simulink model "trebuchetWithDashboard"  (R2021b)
settings: Solver=VariableStepAuto  StartTime=0.0  StopTime=10.0  MaxStep=1e-4  RelTol=1e-4  AbsTol=1e-5
model workspace (MAT data in the model file):
  alpha0 = 0.920523020141
  finang = 19.6743276335
  lsling = 20
  ppos = 3
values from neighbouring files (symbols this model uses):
  in = repmat(Simulink.SimulationInput(mdl),N,1)    [simulateMultipleTrebuchet.m]    (also in simulateTrebuchet.m = in.setVariable('finang',launchAngle,'workspace',mdl))
  N = 20    [simulateMultipleTrebuchet.m]
undefined symbols (not defined in the file or in its folder): deg, ft, kg, lbm, m, s, X, Y, Z
libraries: sm_lib x33, nesl_utility x6, simulink x1

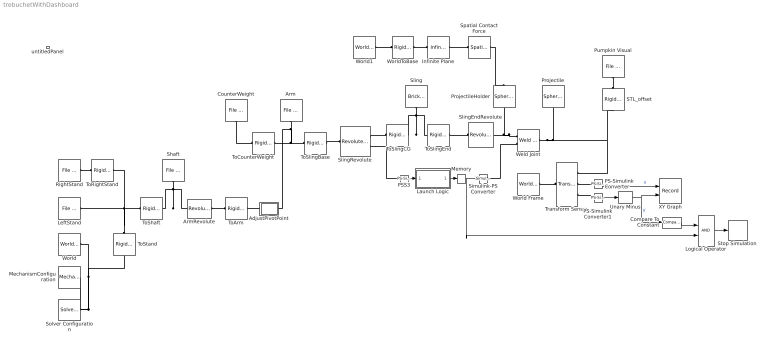
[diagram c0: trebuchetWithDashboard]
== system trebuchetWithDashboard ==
  AdjustPivotPoint : Subsystem
  Arm : sm_lib/Body Elements/File Solid  ExtGeomFileName=arm_prt.stl  UnitType=Custom  ExtGeomFileUnits=in  StepReaderType=HEX  ExportConvexHullGeometry=off  InertiaType=Custom  Mass=1.6  MassUnits=lbm  CenterOfMass=[2.01944889092782 0.231390262424323 -1.93537039141591e-10]  CenterOfMassUnits=in  MomentsOfInertia=[1.99947648053387 238.440492059946 240.01438453116]  MomentsOfInertiaUnits=lbm*in^2  ProductsOfInertia=[0 0 0]  ProductsOfInertiaUnits=lbm*in^2  BasedOnType=Density  Density=800  DensityUnits=kg/(m^3)  DoExposeReferenceFrame=on  SerializedFrames=<Frames/>  GraphicType=FromGeometry  MarkerShape=Sphere  MarkerSize=10  MarkerSizeUnits=m  GraphicVisPropType=SimpleVisualProperties  GraphicDiffuseColor="[0.7137    0.6078    0.2980]"  GraphicSpecularColor=[0.5 0.5 0.5 1.0]  GraphicAmbientColor=[0.15 0.15 0.15 1.0]  GraphicEmissiveColor=[0.0 0.0 0.0 1.0]  GraphicShininess=75  GraphicOpacity=1.0
  ArmRevolute : sm_lib/Joints/Revolute Joint  JointMode=Normal  SenseConstraintForce=off  SenseConstraintForceX=off  SenseConstraintForceY=off  SenseConstraintForceZ=off  SenseConstraintTorque=off  SenseConstraintTorqueX=off  SenseConstraintTorqueY=off  SenseConstraintTorqueZ=off  SenseTotalForce=off  SenseTotalForceX=off  SenseTotalForceY=off  SenseTotalForceZ=off  SenseTotalTorque=off  SenseTotalTorqueX=off  SenseTotalTorqueY=off  SenseTotalTorqueZ=off  CompositeWrenchDir=FollowerOnBase  CompositeWrenchFrame=BaseFrame  EquilibriumPosition=0  EquilibriumPositionUnits=deg  SpringStiffness=0  SpringStiffnessUnits=N*m/deg  DampingCoefficient=0  DampingCoefficientUnits=N*m/(deg/s)  TorqueActuationMode=NoTorque  MotionActuationMode=ComputedMotion  SensePosition=off  SenseVelocity=off  SenseAcceleration=off  SenseTorqueForce=off  SenseLowerLimitTorqueForce=off  SenseUpperLimitTorqueForce=off  LowerLimitSpecify=off  LowerLimitBound=-90  LowerLimitBoundUnits=deg  LowerLimitStiffness=1e4  LowerLimitStiffnessUnits=N*m/deg  LowerLimitDamping=10  LowerLimitDampingUnits=N*m/(deg/s)  LowerLimitTransitionRegionWidth=0.1  LowerLimitTransitionRegionWidthUnits=deg  UpperLimitSpecify=off  UpperLimitBound=90  UpperLimitBoundUnits=deg  UpperLimitStiffness=1e4  UpperLimitStiffnessUnits=N*m/deg  UpperLimitDamping=10  UpperLimitDampingUnits=N*m/(deg/s)  UpperLimitTransitionRegionWidth=0.1  UpperLimitTransitionRegionWidthUnits=deg  PositionTargetSpecify=on  PositionTargetPriority=High  PositionTargetValue=alpha0  PositionTargetValueUnits=rad  VelocityTargetSpecify=off  VelocityTargetPriority=High  VelocityTargetValue=0  VelocityTargetValueUnits=deg/s
  Compare To Constant : simulink/Logic and Bit Operations/Compare To Constant  relop=<=  const=-0.1  OutDataTypeStr=boolean
  CounterWeight : sm_lib/Body Elements/File Solid  ExtGeomFileName=cweight_prt.stl  UnitType=Custom  ExtGeomFileUnits=in  StepReaderType=HEX  ExportConvexHullGeometry=off  InertiaType=Custom  Mass=20  MassUnits=lbm  CenterOfMass=[0 0 0]  CenterOfMassUnits=in  MomentsOfInertia=[180.271839940582 180.271699524682 219.335621261554]  MomentsOfInertiaUnits=lbm*in^2  ProductsOfInertia=[0 0 0]  ProductsOfInertiaUnits=lbm*in^2  BasedOnType=Density  Density=8200  DensityUnits=kg/(m^3)  DoExposeReferenceFrame=on  SerializedFrames=<Frames/>  GraphicType=FromGeometry  MarkerShape=Sphere  MarkerSize=10  MarkerSizeUnits=m  GraphicVisPropType=SimpleVisualProperties  GraphicDiffuseColor=[0.5 0.5 0.5]  GraphicSpecularColor=[0.5 0.5 0.5 1.0]  GraphicAmbientColor=[0.15 0.15 0.15 1.0]  GraphicEmissiveColor=[0.0 0.0 0.0 1.0]  GraphicShininess=75  GraphicOpacity=1.0
  Infinite Plane : sm_lib/Curves and Surfaces/Infinite Plane  GraphicType=Rectangle  GraphicPlaneWidth=5  GraphicPlaneWidthUnits=m  GraphicPlaneHeight=5  GraphicPlaneHeightUnits=m  GraphicVisPropType=SimpleVisualProperties  GraphicDiffuseColor=[1 1 1]  GraphicOpacity=0.25  GraphicSpecularColor=[0.5 0.5 0.5 1.0]  GraphicAmbientColor=[0.15 0.15 0.15 1.0]  GraphicEmissiveColor=[0.0 0.0 0.0 1.0]  GraphicShininess=75
  Launch Logic : Stateflow chart  TreatAsAtomicUnit=on
  LeftStand : sm_lib/Body Elements/File Solid  ExtGeomFileName=upright_prt.stl  UnitType=Custom  ExtGeomFileUnits=in  StepReaderType=HEX  ExportConvexHullGeometry=off  InertiaType=Custom  Mass=5  MassUnits=lbm  CenterOfMass=[0 -6.3095100000000004 0.38968399999999997]  CenterOfMassUnits=in  MomentsOfInertia=[11765.6 43021.699999999997 54038.900000000001]  MomentsOfInertiaUnits=lbm*in^2  ProductsOfInertia=[1161.4200000000001 0 0]  ProductsOfInertiaUnits=lbm*in^2  BasedOnType=Density  Density=1000  DensityUnits=kg/(m^3)  DoExposeReferenceFrame=on  SerializedFrames=<Frames/>  GraphicType=FromGeometry  MarkerShape=Sphere  MarkerSize=10  MarkerSizeUnits=m  GraphicVisPropType=SimpleVisualProperties  GraphicDiffuseColor="[0.5098    0.3216    0.0039]"  GraphicSpecularColor=[0.5 0.5 0.5 1.0]  GraphicAmbientColor=[0.15 0.15 0.15 1.0]  GraphicEmissiveColor=[0.0 0.0 0.0 1.0]  GraphicShininess=75  GraphicOpacity=0.2
  Logical Operator : Logic  AllPortsSameDT=off  OutDataTypeStr=boolean
  MechanismConfiguration : sm_lib/Utilities/Mechanism Configuration  UniformGravity=Constant  GravityVector=[0 32.174 0]  GravityUnits=ft/s^2  LinearizationDelta=0.001  JointModeTransitionNonlinearIterations=2
  Memory : Memory
  PS-Simulink Converter : nesl_utility/PS-Simulink Converter  PhysicalDomain=network_engine_domain  SubClassName=ps_output  LeftPortType=input  RightPortType=output  PseudoPeriodic=off  Frequencies=[]  Unit=inherit  AffineConversion=off
  PS-Simulink Converter1 : nesl_utility/PS-Simulink Converter  PhysicalDomain=network_engine_domain  SubClassName=ps_output  LeftPortType=input  RightPortType=output  PseudoPeriodic=off  Frequencies=[]  Unit=inherit  AffineConversion=off
  PSS3 : nesl_utility/PS-Simulink Converter  PhysicalDomain=network_engine_domain  SubClassName=ps_output  LeftPortType=input  RightPortType=output  PseudoPeriodic=off  Frequencies=[]  Unit=deg  AffineConversion=off
  Projectile : sm_lib/Body Elements/Spherical Solid  GraphicAmbientColor=[0.15 0.15 0.15 1.0]  BasedOnType=Density  CenterOfMass=[0 0 0]  CenterOfMassUnits=m  GraphicDiffuseColor=[0.4 1.0 0.4]  Density=3000*10  DensityUnits=kg/m^3  DoExposeReferenceFrame=on  GraphicEmissiveColor=[0.0 0.0 0.0 1.0]  ExportEntireGeometry=off  SerializedExposedGeometries=<ExposedGeometries/>  SerializedFrames=<Frames/>  MarkerShape=Sphere  MarkerSize=10  GraphicType=FromGeometry  InertiaType=CalculateFromGeometry  Mass=0.074  MassUnits=lbm  MomentsOfInertia=[1 1 1]  MomentsOfInertiaUnits=lbm*in^2  GraphicOpacity=0.2  ProductsOfInertia=[0 0 0]  ProductsOfInertiaUnits=lbm*in^2  GraphicShininess=75  GraphicSpecularColor=[0.5 0.5 0.5 1.0]  SphereRadius=0.624  SphereRadiusUnits=in  GraphicVisPropType=SimpleVisualProperties
  ProjectileHolder : sm_lib/Body Elements/Spherical Solid  GraphicAmbientColor=[0.15 0.15 0.15 1.0]  BasedOnType=Density  CenterOfMass=[0 0 0]  CenterOfMassUnits=m  GraphicDiffuseColor=[1 0.25 0]  Density=3000  DensityUnits=kg/m^3  DoExposeReferenceFrame=on  GraphicEmissiveColor=[0.0 0.0 0.0 1.0]  ExportEntireGeometry=on  SerializedExposedGeometries=<ExposedGeometries><ExposedGeometry><RawGeometryId>entire</RawGeometryId><ExposedGeometryId>G</ExposedGeometryId></ExposedGeometry></ExposedGeometries>  SerializedFrames=<Frames/>  MarkerShape=Sphere  MarkerSize=10  GraphicType=FromGeometry  InertiaType=Custom  Mass=0.001  MassUnits=kg  MomentsOfInertia=[1 1 1]  MomentsOfInertiaUnits=lbm*in^2  GraphicOpacity=1.0  ProductsOfInertia=[0 0 0]  ProductsOfInertiaUnits=lbm*in^2  GraphicShininess=75  GraphicSpecularColor=[0.5 0.5 0.5 1.0]  SphereRadius=0.624  SphereRadiusUnits=in  GraphicVisPropType=SimpleVisualProperties
  Pumpkin Visual : sm_lib/Body Elements/File Solid  ExtGeomFileName=pumpkinskull_earring_remix.stl  UnitType=Custom  ExtGeomFileUnits=cm  StepReaderType=HEX  ExportConvexHullGeometry=off  InertiaType=PointMass  Mass=0  MassUnits=kg  CenterOfMass=[0 0 0]  CenterOfMassUnits=m  MomentsOfInertia=[1 1 1]  MomentsOfInertiaUnits=kg*m^2  ProductsOfInertia=[0 0 0]  ProductsOfInertiaUnits=kg*m^2  BasedOnType=DensityFromFile  Density=1000  DensityUnits=kg/m^3  DoExposeReferenceFrame=on  SerializedFrames=<Frames/>  GraphicType=FromGeometry  MarkerShape=Sphere  MarkerSize=10  GraphicVisPropType=SimpleVisualProperties  GraphicDiffuseColor=[1.0 0.4 0.0]  GraphicSpecularColor=[0.5 0.5 0.5 1.0]  GraphicAmbientColor=[0.15 0.15 0.15 1.0]  GraphicEmissiveColor=[0.0 0.0 0.0 1.0]  GraphicShininess=75  GraphicOpacity=1.0
  RightStand : sm_lib/Body Elements/File Solid  ExtGeomFileName=prt0002_prt.stl  UnitType=Custom  ExtGeomFileUnits=in  StepReaderType=HEX  ExportConvexHullGeometry=off  InertiaType=Custom  Mass=5  MassUnits=lbm  CenterOfMass=[0 -6.3095100000000004 -0.38968399999999997]  CenterOfMassUnits=in  MomentsOfInertia=[11765.6 43021.699999999997 54038.900000000001]  MomentsOfInertiaUnits=lbm*in^2  ProductsOfInertia=[-1161.4200000000001 0 0]  ProductsOfInertiaUnits=lbm*in^2  BasedOnType=Density  Density=1000  DensityUnits=kg/(m^3)  DoExposeReferenceFrame=on  SerializedFrames=<Frames/>  GraphicType=FromGeometry  MarkerShape=Sphere  MarkerSize=10  MarkerSizeUnits=m  GraphicVisPropType=SimpleVisualProperties  GraphicDiffuseColor="[0.5098    0.3216    0.0039]"  GraphicSpecularColor=[0.5 0.5 0.5 1.0]  GraphicAmbientColor=[0.15 0.15 0.15 1.0]  GraphicEmissiveColor=[0.0 0.0 0.0 1.0]  GraphicShininess=75  GraphicOpacity=0.2
  STL_offset : sm_lib/Frames and Transforms/Rigid Transform  TranslationMethod=Cartesian  TranslationStandardOffset=0  TranslationLengthUnit=m  TranslationStandardAxis=+Z  TranslationCartesianOffset=[-1 0 1]  TranslationROffset=0  TranslationROffsetUnits=m  TranslationZOffset=0  TranslationZOffsetUnits=m  TranslationThetaOffset=0  TranslationThetaOffsetUnits=deg  RotationMethod=StandardAxis  RotationAngleUnits=deg  RotationStandardAxis=+X  RotationAngle=-90  RotationArbitraryAxis=[0 0 1]  FollAlignAxisA=+X  BaseAlignAxisA=+Y  FollAlignAxisB=+Y  BaseAlignAxisB=+Z  RotationSequenceAxes=FollowerAxes  RotationSequence=XYX  RotationSequenceAngles=[0 0 0]  RotationSequenceAnglesUnits=deg  RotationMatrix=[1 0 0; 0 1 0; 0 0 1]
  Shaft : sm_lib/Body Elements/File Solid  ExtGeomFileName=shaft1_prt.stl  UnitType=Custom  ExtGeomFileUnits=in  StepReaderType=HEX  ExportConvexHullGeometry=off  InertiaType=Custom  Mass=0.75161  MassUnits=lbm  CenterOfMass=[0 -1.44250608133824e-19 -3.11581313569059e-16]  CenterOfMassUnits=in  MomentsOfInertia=[6.64610546204847 6.64664045415189 0.039282600271159]  MomentsOfInertiaUnits=lbm*in^2  ProductsOfInertia=[0 0 0]  ProductsOfInertiaUnits=lbm*in^2  BasedOnType=Density  Density=7850  DensityUnits=kg/(m^3)  DoExposeReferenceFrame=on  SerializedFrames=<Frames/>  GraphicType=FromGeometry  MarkerShape=Sphere  MarkerSize=10  MarkerSizeUnits=m  GraphicVisPropType=SimpleVisualProperties  GraphicDiffuseColor=[0.5 0.5 0.5]  GraphicSpecularColor=[0.5 0.5 0.5 1.0]  GraphicAmbientColor=[0.15 0.15 0.15 1.0]  GraphicEmissiveColor=[0.0 0.0 0.0 1.0]  GraphicShininess=75  GraphicOpacity=1.0
  Simulink-PS Converter : nesl_utility/Simulink-PS Converter  PhysicalDomain=network_engine_domain  SubClassName=ps_input  LeftPortType=input  RightPortType=output  PseudoPeriodic=off  Frequencies=[]  NoiseDistribution=none  NoiseParameters=[]  Unit=1  AffineConversion=off  FilteringAndDerivatives=provide  SimscapeFilterOrder=1  InputFilterTimeConstant=0.001  UdotUserProvided=0
  Sling : sm_lib/Body Elements/Brick Solid  GraphicAmbientColor=[0.15 0.15 0.15 1.0]  BasedOnType=Density  BrickDimensions=[lsling .05 .05]  BrickDimensionUnits=in  CenterOfMass=[0 0 0]  CenterOfMassUnits=m  GraphicDiffuseColor=[0.0 0 0.0]  Density=1  DensityUnits=kg/(m^3)  DoExposeReferenceFrame=on  GraphicEmissiveColor=[0.0 0.0 0.0 1.0]  ExportEntireGeometry=off  SerializedFrames=<Frames/>  MarkerShape=Sphere  MarkerSize=10  GraphicType=FromGeometry  InertiaType=CalculateFromGeometry  Mass=1  MassUnits=kg  MomentsOfInertia=[1 1 1]  MomentsOfInertiaUnits=kg*m^2  GraphicOpacity=1.0  ProductsOfInertia=[0 0 0]  ProductsOfInertiaUnits=kg*m^2  GraphicShininess=75  GraphicSpecularColor=[0.5 0.5 0.5 1.0]  GraphicVisPropType=SimpleVisualProperties
  SlingEndRevolute : sm_lib/Joints/Revolute Joint  JointMode=Normal  SenseConstraintForce=off  SenseConstraintForceX=off  SenseConstraintForceY=off  SenseConstraintForceZ=off  SenseConstraintTorque=off  SenseConstraintTorqueX=off  SenseConstraintTorqueY=off  SenseConstraintTorqueZ=off  SenseTotalForce=off  SenseTotalForceX=off  SenseTotalForceY=off  SenseTotalForceZ=off  SenseTotalTorque=off  SenseTotalTorqueX=off  SenseTotalTorqueY=off  SenseTotalTorqueZ=off  CompositeWrenchDir=FollowerOnBase  CompositeWrenchFrame=BaseFrame  EquilibriumPosition=0  EquilibriumPositionUnits=deg  SpringStiffness=0  SpringStiffnessUnits=N*m/deg  DampingCoefficient=0  DampingCoefficientUnits=N*m/(deg/s)  TorqueActuationMode=NoTorque  MotionActuationMode=ComputedMotion  SensePosition=off  SenseVelocity=off  SenseAcceleration=off  SenseTorqueForce=off  SenseLowerLimitTorqueForce=off  SenseUpperLimitTorqueForce=off  LowerLimitSpecify=off  LowerLimitBound=-90  LowerLimitBoundUnits=deg  LowerLimitStiffness=1e4  LowerLimitStiffnessUnits=N*m/deg  LowerLimitDamping=10  LowerLimitDampingUnits=N*m/(deg/s)  LowerLimitTransitionRegionWidth=0.1  LowerLimitTransitionRegionWidthUnits=deg  UpperLimitSpecify=off  UpperLimitBound=90  UpperLimitBoundUnits=deg  UpperLimitStiffness=1e4  UpperLimitStiffnessUnits=N*m/deg  UpperLimitDamping=10  UpperLimitDampingUnits=N*m/(deg/s)  UpperLimitTransitionRegionWidth=0.1  UpperLimitTransitionRegionWidthUnits=deg  PositionTargetSpecify=off  PositionTargetPriority=High  PositionTargetValue=-48.6  PositionTargetValueUnits=deg  VelocityTargetSpecify=off  VelocityTargetPriority=High  VelocityTargetValue=0  VelocityTargetValueUnits=deg/s
  SlingRevolute : sm_lib/Joints/Revolute Joint  JointMode=Normal  SenseConstraintForce=off  SenseConstraintForceX=off  SenseConstraintForceY=off  SenseConstraintForceZ=off  SenseConstraintTorque=off  SenseConstraintTorqueX=off  SenseConstraintTorqueY=off  SenseConstraintTorqueZ=off  SenseTotalForce=off  SenseTotalForceX=off  SenseTotalForceY=off  SenseTotalForceZ=off  SenseTotalTorque=off  SenseTotalTorqueX=off  SenseTotalTorqueY=off  SenseTotalTorqueZ=off  CompositeWrenchDir=FollowerOnBase  CompositeWrenchFrame=BaseFrame  EquilibriumPosition=0  EquilibriumPositionUnits=deg  SpringStiffness=0  SpringStiffnessUnits=N*m/deg  DampingCoefficient=0  DampingCoefficientUnits=N*m/(deg/s)  TorqueActuationMode=NoTorque  MotionActuationMode=ComputedMotion  SensePosition=on  SenseVelocity=off  SenseAcceleration=off  SenseTorqueForce=off  SenseLowerLimitTorqueForce=off  SenseUpperLimitTorqueForce=off  LowerLimitSpecify=off  LowerLimitBound=-90  LowerLimitBoundUnits=deg  LowerLimitStiffness=1e4  LowerLimitStiffnessUnits=N*m/deg  LowerLimitDamping=10  LowerLimitDampingUnits=N*m/(deg/s)  LowerLimitTransitionRegionWidth=0.1  LowerLimitTransitionRegionWidthUnits=deg  UpperLimitSpecify=off  UpperLimitBound=90  UpperLimitBoundUnits=deg  UpperLimitStiffness=1e4  UpperLimitStiffnessUnits=N*m/deg  UpperLimitDamping=10  UpperLimitDampingUnits=N*m/(deg/s)  UpperLimitTransitionRegionWidth=0.1  UpperLimitTransitionRegionWidthUnits=deg  PositionTargetSpecify=on  PositionTargetPriority=High  PositionTargetValue=-35  PositionTargetValueUnits=deg  VelocityTargetSpecify=off  VelocityTargetPriority=High  VelocityTargetValue=0  VelocityTargetValueUnits=deg/s
  Solver Configuration : nesl_utility/Solver Configuration  PhysicalDomain=network_engine_domain  SubClassName=solver  LeftPortType=input  RightPortType=generic  Tones=[]  Harmonics=[]  SimulateNoise=off  Profile=off  UseLocalSampling=off  EnableSwitchedLinearOptims=on  FrequencyDomain=off  UseCCode=off  RelTol=0.001  AbsTol=1e-06  MinStep=1e-09  ToWorkspace=off  RevertToSquareIcSolve=off  NumHomotopyIterations=100  PhasorMode=off  PhasorModeNumHarmonics=1  DoDC=off  ResidualTolerance=1e-9  UseLocalSolver=off  LocalSolverChoice=NE_BACKWARD_EULER_ADVANCER  LocalSolverSampleTime=.001  DoFixedCost=off  MaxNonlinIter=3  MaxModeIter=2  ComputeImpulses=off  ImpulseIterations=2  LinearAlgebra=Sparse  EquationFormulation=NE_TIME_EF  DelaysMemoryBudget=1024  AutomaticFiltering=on  FilteringTimeConstant=0.001  PartitionStorageMethod=AS_NEEDED  PartitionMemoryBudget=1024  PartitionMethod=FAST
  Spatial Contact Force : sm_lib/Forces and Torques/Spatial Contact Force  CoefficientOfDynamicFriction=0.3  CoefficientOfStaticFriction=0.5  SenseContactBaseRotation=off  SenseContactBaseTranslation=off  NormalDamping=1e3  NormalDampingUnits=N/(m/s)  SenseContactFollowerRotation=off  SenseContactFollowerTranslation=off  SenseContactSignal=off  NormalStiffness=1e6  NormalStiffnessUnits=N/m  FrictionalCriticalVelocity=1e-3  FrictionalCriticalVelocityUnits=m/s  ZeroCrossDetectContactStartAndEnd=on  FrictionType=None  SenseFrictionalForceMagnitude=off  SenseNormalForceMagnitude=off  NormalForceType=SmoothSpringDamper  SenseNormalVelocity=off  SenseSeparationDistance=off  SenseTangentialVelocity=off  SenseTangentialVelocityMagnitude=off  NormalTransitionRegionWidth=1e-4  NormalTransitionRegionWidthUnits=m
  Stop Simulation : Stop
  ToArm : sm_lib/Frames and Transforms/Rigid Transform  TranslationMethod=StandardAxis  TranslationStandardOffset=ppos  TranslationLengthUnit=in  TranslationStandardAxis=+X  TranslationCartesianOffset=[16.25 0 0.5]  TranslationROffset=0  TranslationROffsetUnits=m  TranslationZOffset=0  TranslationZOffsetUnits=m  TranslationThetaOffset=0  TranslationThetaOffsetUnits=deg  RotationMethod=None  RotationAngleUnits=rad  RotationStandardAxis=+Z  RotationAngle=0  RotationArbitraryAxis=[0 0 0]  FollAlignAxisA=+X  BaseAlignAxisA=+Y  FollAlignAxisB=+Y  BaseAlignAxisB=+Z  RotationSequenceAxes=FollowerAxes  RotationSequence=XYX  RotationSequenceAngles=[0 0 0]  RotationSequenceAnglesUnits=deg  RotationMatrix=[1 0 0; 0 1 0; 0 0 1]
  ToCounterWeight : sm_lib/Frames and Transforms/Rigid Transform  TranslationMethod=Cartesian  TranslationStandardOffset=0  TranslationLengthUnit=in  TranslationStandardAxis=+Z  TranslationCartesianOffset=[0 0 0.52167589999999997]-[16.25 0 0.5]  TranslationROffset=0  TranslationROffsetUnits=m  TranslationZOffset=0  TranslationZOffsetUnits=m  TranslationThetaOffset=0  TranslationThetaOffsetUnits=deg  RotationMethod=ArbitraryAxis  RotationAngleUnits=rad  RotationStandardAxis=+Z  RotationAngle=0  RotationArbitraryAxis=[0 0 0]  FollAlignAxisA=+X  BaseAlignAxisA=+Y  FollAlignAxisB=+Y  BaseAlignAxisB=+Z  RotationSequenceAxes=FollowerAxes  RotationSequence=XYX  RotationSequenceAngles=[0 0 0]  RotationSequenceAnglesUnits=deg  RotationMatrix=[1 0 0; 0 1 0; 0 0 1]
  ToRightStand : sm_lib/Frames and Transforms/Rigid Transform  TranslationMethod=Cartesian  TranslationStandardOffset=0  TranslationLengthUnit=in  TranslationStandardAxis=+Z  TranslationCartesianOffset=[57.600000000000001 11 -9.25]-[57.600000000000001 11 -2]  TranslationROffset=0  TranslationROffsetUnits=m  TranslationZOffset=0  TranslationZOffsetUnits=m  TranslationThetaOffset=0  TranslationThetaOffsetUnits=deg  RotationMethod=None  RotationAngleUnits=deg  RotationStandardAxis=+Z  RotationAngle=0  RotationArbitraryAxis=[0 0 1]  FollAlignAxisA=+X  BaseAlignAxisA=+Y  FollAlignAxisB=+Y  BaseAlignAxisB=+Z  RotationSequenceAxes=FollowerAxes  RotationSequence=XYX  RotationSequenceAngles=[0 0 0]  RotationSequenceAnglesUnits=deg  RotationMatrix=[1 0 0; 0 1 0; 0 0 1]
  ToShaft : sm_lib/Frames and Transforms/Rigid Transform  TranslationMethod=Cartesian  TranslationStandardOffset=0  TranslationLengthUnit=in  TranslationStandardAxis=+Z  TranslationCartesianOffset=[0 9 0]-[0 0 3.625]  TranslationROffset=0  TranslationROffsetUnits=m  TranslationZOffset=0  TranslationZOffsetUnits=m  TranslationThetaOffset=0  TranslationThetaOffsetUnits=deg  RotationMethod=ArbitraryAxis  RotationAngleUnits=rad  RotationStandardAxis=+Z  RotationAngle=0  RotationArbitraryAxis=[0 0 0]  FollAlignAxisA=+X  BaseAlignAxisA=+Y  FollAlignAxisB=+Y  BaseAlignAxisB=+Z  RotationSequenceAxes=FollowerAxes  RotationSequence=XYX  RotationSequenceAngles=[0 0 0]  RotationSequenceAnglesUnits=deg  RotationMatrix=[1 0 0; 0 1 0; 0 0 1]
  ToSlingBase : sm_lib/Frames and Transforms/Rigid Transform  TranslationMethod=Cartesian  TranslationStandardOffset=0  TranslationLengthUnit=in  TranslationStandardAxis=+Z  TranslationCartesianOffset=[-17.75 0 0]  TranslationROffset=0  TranslationROffsetUnits=m  TranslationZOffset=0  TranslationZOffsetUnits=m  TranslationThetaOffset=0  TranslationThetaOffsetUnits=deg  RotationMethod=ArbitraryAxis  RotationAngleUnits=rad  RotationStandardAxis=+Z  RotationAngle=0  RotationArbitraryAxis=[0 0 0]  FollAlignAxisA=+X  BaseAlignAxisA=+Y  FollAlignAxisB=+Y  BaseAlignAxisB=+Z  RotationSequenceAxes=FollowerAxes  RotationSequence=XYX  RotationSequenceAngles=[0 0 0]  RotationSequenceAnglesUnits=deg  RotationMatrix=[1 0 0; 0 1 0; 0 0 1]
  ToSlingCG : sm_lib/Frames and Transforms/Rigid Transform  TranslationMethod=StandardAxis  TranslationStandardOffset=lsling/2  TranslationLengthUnit=in  TranslationStandardAxis=+X  TranslationCartesianOffset=[0 0 0]  TranslationROffset=0  TranslationROffsetUnits=m  TranslationZOffset=0  TranslationZOffsetUnits=m  TranslationThetaOffset=0  TranslationThetaOffsetUnits=deg  RotationMethod=None  RotationAngleUnits=deg  RotationStandardAxis=+Z  RotationAngle=0  RotationArbitraryAxis=[0 0 1]  FollAlignAxisA=+X  BaseAlignAxisA=+Y  FollAlignAxisB=+Y  BaseAlignAxisB=+Z  RotationSequenceAxes=FollowerAxes  RotationSequence=XYX  RotationSequenceAngles=[0 0 0]  RotationSequenceAnglesUnits=deg  RotationMatrix=[1 0 0; 0 1 0; 0 0 1]
  ToSlingEnd : sm_lib/Frames and Transforms/Rigid Transform  TranslationMethod=StandardAxis  TranslationStandardOffset=-lsling/2  TranslationLengthUnit=in  TranslationStandardAxis=-X  TranslationCartesianOffset=[0 0 0]  TranslationROffset=0  TranslationROffsetUnits=m  TranslationZOffset=0  TranslationZOffsetUnits=m  TranslationThetaOffset=0  TranslationThetaOffsetUnits=deg  RotationMethod=None  RotationAngleUnits=deg  RotationStandardAxis=+Z  RotationAngle=0  RotationArbitraryAxis=[0 0 1]  FollAlignAxisA=+X  BaseAlignAxisA=+Y  FollAlignAxisB=+Y  BaseAlignAxisB=+Z  RotationSequenceAxes=FollowerAxes  RotationSequence=XYX  RotationSequenceAngles=[0 0 0]  RotationSequenceAnglesUnits=deg  RotationMatrix=[1 0 0; 0 1 0; 0 0 1]
  ToStand : sm_lib/Frames and Transforms/Rigid Transform  TranslationMethod=Cartesian  TranslationStandardOffset=0  TranslationLengthUnit=in  TranslationStandardAxis=+Z  TranslationCartesianOffset=[-18 0 0]  TranslationROffset=0  TranslationROffsetUnits=m  TranslationZOffset=0  TranslationZOffsetUnits=m  TranslationThetaOffset=0  TranslationThetaOffsetUnits=deg  RotationMethod=ArbitraryAxis  RotationAngleUnits=rad  RotationStandardAxis=+Z  RotationAngle=3.1415926535897931  RotationArbitraryAxis=[1 0 0]  FollAlignAxisA=+X  BaseAlignAxisA=+Y  FollAlignAxisB=+Y  BaseAlignAxisB=+Z  RotationSequenceAxes=FollowerAxes  RotationSequence=XYX  RotationSequenceAngles=[0 0 0]  RotationSequenceAnglesUnits=deg  RotationMatrix=[1 0 0; 0 1 0; 0 0 1]
  Transform Sensor : sm_lib/Frames and Transforms/Transform Sensor  MeasurementFrame=World  SenseAngle=off  SenseAxis=off  SenseAngle1=off  SenseAngle2=off  SenseAngle3=off  SenseQ=off  SenseR=off  SenseOmegaX=off  SenseOmegaY=off  SenseOmegaZ=off  SenseOmega1=off  SenseOmega2=off  SenseOmega3=off  SenseQDot=off  SenseRDot=off  SenseAlphaX=off  SenseAlphaY=off  SenseAlphaZ=off  SenseAlpha1=off  SenseAlpha2=off  SenseAlpha3=off  SenseQDDot=off  SenseRDDot=off  SenseX=on  SenseY=on  SenseZ=off  SenseRad=off  SenseAzim=off  SenseDist=off  SenseInc=off  SenseXDot=off  SenseYDot=off  SenseZDot=off  SenseRadDot=off  SenseAzimDot=off  SenseDistDot=off  SenseIncDot=off  SenseXDDot=off  SenseYDDot=off  SenseZDDot=off  SenseRadDDot=off  SenseAzimDDot=off  SenseDistDDot=off  SenseIncDDot=off
  Unary Minus : UnaryMinus
  Weld Joint : sm_lib/Joints/Weld Joint  JointMode=ProvidedByInput  SenseConstraintForce=off  SenseConstraintForceX=off  SenseConstraintForceY=off  SenseConstraintForceZ=off  SenseConstraintTorque=off  SenseConstraintTorqueX=off  SenseConstraintTorqueY=off  SenseConstraintTorqueZ=off  SenseTotalForce=off  SenseTotalForceX=off  SenseTotalForceY=off  SenseTotalForceZ=off  SenseTotalTorque=off  SenseTotalTorqueX=off  SenseTotalTorqueY=off  SenseTotalTorqueZ=off  CompositeWrenchDir=FollowerOnBase  CompositeWrenchFrame=BaseFrame
  World : sm_lib/Frames and Transforms/World Frame
  World Frame : sm_lib/Frames and Transforms/World Frame
  World1 : sm_lib/Frames and Transforms/World Frame
  WorldToBase : sm_lib/Frames and Transforms/Rigid Transform  TranslationMethod=Cartesian  TranslationStandardOffset=0  TranslationLengthUnit=in  TranslationStandardAxis=+Z  TranslationCartesianOffset=[18 11.375 3.625]  TranslationROffset=0  TranslationROffsetUnits=m  TranslationZOffset=0  TranslationZOffsetUnits=m  TranslationThetaOffset=0  TranslationThetaOffsetUnits=deg  RotationMethod=StandardAxis  RotationAngleUnits=deg  RotationStandardAxis=+X  RotationAngle=90  RotationArbitraryAxis=[-1 0 0]  FollAlignAxisA=+X  BaseAlignAxisA=+Y  FollAlignAxisB=+Y  BaseAlignAxisB=+Z  RotationSequenceAxes=FollowerAxes  RotationSequence=XYX  RotationSequenceAngles=[0 0 0]  RotationSequenceAnglesUnits=deg  RotationMatrix=[1 0 0; 0 1 0; 0 0 1]
  XY Graph : Record  FileSettingsInternal="{\"entries\":[{\"content\":{\"excelSettings\":{\"content\":{},\"type\":\"Streamout.ExcelSettings\"}},\"type\":\"Streamout.FileSettingStorage\",\"uuid\":\"d316082e-d6c1-4aab-8ad4-36e511cd561d\"}],\"packageUris\":[\"http://schema.mathworks.com/mf0/streamout_blocks/R2020a\"],\"version\":\"1.0\"}"  Layout=[1 1]  SignalsInternal="{\"entries\":[{\"content\":{\"signals\":[{\"content\":{\"blockPath\":[\"trebuchetWithDashboard/XY Graph\"],\"channel\":[],\"dimensions\":[1],\"domain\":\"trebuchetWithDashboard/XY Graph\",\"lineColor\":\"#7e2f8e\",\"plots\":[],\"port\":1,\"sid\":[],\"signalID\":26672,\"signalName\":\"x\"},\"type\":\"RecordBlkView.Signal\",\"uuid\":\"8ffd9437-4e01-4f17-9f1d-eb5391d8b48f\"},{\"content\":{\"blockPath\":[\"trebuchetWithDashboard/XY Graph\"],\"channel\"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"  VisualizationBindings="{\"xyplotplugin\":{\"info\":[{\"series\":[],\"subplotID\":1}]}}"  CompatibilityTag=XY
  untitledPanel : Subsystem  Tag=HiddenForWebPanel  IsWebBlockPanel=on
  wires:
  PS-Simulink Converter1/1 -> Unary Minus/1
  Launch Logic/1(mode) -> Memory/1
  Memory/1 -> Logical Operator/2, Simulink-PS Converter/1
  Logical Operator/1 -> Stop Simulation/1
  Compare To Constant/1 -> Logical Operator/1
  PSS3/1 -> Launch Logic/1(u)
  PS-Simulink Converter/1 -> XY Graph/1  "x"
  Unary Minus/1 -> XY Graph/2, Compare To Constant/1  "y"
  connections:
  Sling/RConn1 -- ToSlingEnd/LConn1 -- ToSlingCG/RConn1
  Arm/RConn1 -- ToSlingBase/LConn1 -- AdjustPivotPoint/RConn1 -- ToCounterWeight/RConn1
  ToStand/LConn1 -- ToShaft/LConn1 -- ToRightStand/LConn1 -- LeftStand/RConn1
  Weld Joint/RConn1 -- Projectile/RConn1 -- Transform Sensor/RConn1 -- STL_offset/LConn1
  Weld Joint/LConn1 -- ProjectileHolder/RConn1 -- SlingEndRevolute/RConn1
  Shaft/RConn1 -- ArmRevolute/LConn1 -- ToShaft/RConn1
  Solver Configuration/RConn1 -- MechanismConfiguration/RConn1 -- ToStand/RConn1 -- World/RConn1
  ToArm/RConn1 -- ArmRevolute/RConn1
  PS-Simulink Converter1/LConn1 -- Transform Sensor/RConn3
  Spatial Contact Force/RConn1 -- ProjectileHolder/LConn1
  ToArm/LConn1 -- AdjustPivotPoint/LConn1
  PSS3/LConn1 -- SlingRevolute/RConn2
  STL_offset/RConn1 -- Pumpkin Visual/RConn1
  World Frame/RConn1 -- Transform Sensor/LConn1
  SlingRevolute/RConn1 -- ToSlingCG/LConn1
  CounterWeight/RConn1 -- ToCounterWeight/LConn1
  SlingEndRevolute/LConn1 -- ToSlingEnd/RConn1
  Transform Sensor/RConn2 -- PS-Simulink Converter/LConn1
  Simulink-PS Converter/RConn1 -- Weld Joint/LConn2
  WorldToBase/LConn1 -- World1/RConn1
  Spatial Contact Force/LConn1 -- Infinite Plane/RConn1
  WorldToBase/RConn1 -- Infinite Plane/LConn1
  ToSlingBase/RConn1 -- SlingRevolute/LConn1
  ToRightStand/RConn1 -- RightStand/RConn1

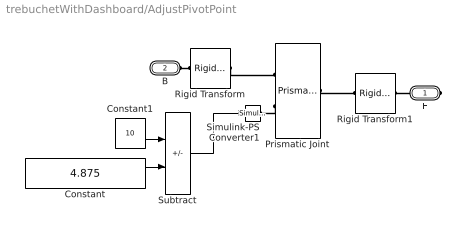
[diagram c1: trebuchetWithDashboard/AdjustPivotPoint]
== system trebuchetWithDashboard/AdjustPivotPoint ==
  Constant : Constant  Value=4.875
  Constant1 : Constant  Value=10
  Prismatic Joint : sm_lib/Joints/Prismatic Joint  JointMode=Normal  SenseConstraintForce=off  SenseConstraintForceX=off  SenseConstraintForceY=off  SenseConstraintForceZ=off  SenseConstraintTorque=off  SenseConstraintTorqueX=off  SenseConstraintTorqueY=off  SenseConstraintTorqueZ=off  SenseTotalForce=off  SenseTotalForceX=off  SenseTotalForceY=off  SenseTotalForceZ=off  SenseTotalTorque=off  SenseTotalTorqueX=off  SenseTotalTorqueY=off  SenseTotalTorqueZ=off  CompositeWrenchDir=FollowerOnBase  CompositeWrenchFrame=BaseFrame  EquilibriumPosition=0  EquilibriumPositionUnits=m  SpringStiffness=0  SpringStiffnessUnits=N/m  DampingCoefficient=0  DampingCoefficientUnits=N/(m/s)  TorqueActuationMode=ComputedTorque  MotionActuationMode=InputMotion  SensePosition=off  SenseVelocity=off  SenseAcceleration=off  SenseTorqueForce=off  SenseLowerLimitTorqueForce=off  SenseUpperLimitTorqueForce=off  LowerLimitSpecify=off  LowerLimitBound=-1  LowerLimitBoundUnits=m  LowerLimitStiffness=1e6  LowerLimitStiffnessUnits=N/m  LowerLimitDamping=1e3  LowerLimitDampingUnits=N/(m/s)  LowerLimitTransitionRegionWidth=1e-4  LowerLimitTransitionRegionWidthUnits=m  UpperLimitSpecify=off  UpperLimitBound=1  UpperLimitBoundUnits=m  UpperLimitStiffness=1e6  UpperLimitStiffnessUnits=N/m  UpperLimitDamping=1e3  UpperLimitDampingUnits=N/(m/s)  UpperLimitTransitionRegionWidth=1e-4  UpperLimitTransitionRegionWidthUnits=m  PositionTargetSpecify=off  PositionTargetPriority=High  PositionTargetValue=0  PositionTargetValueUnits=m  VelocityTargetSpecify=off  VelocityTargetPriority=High  VelocityTargetValue=0  VelocityTargetValueUnits=m/s
  Rigid Transform : sm_lib/Frames and Transforms/Rigid Transform  TranslationMethod=None  TranslationStandardOffset=0  TranslationLengthUnit=m  TranslationStandardAxis=+Z  TranslationCartesianOffset=[0 0 0]  TranslationROffset=0  TranslationROffsetUnits=m  TranslationZOffset=0  TranslationZOffsetUnits=m  TranslationThetaOffset=0  TranslationThetaOffsetUnits=deg  RotationMethod=StandardAxis  RotationAngleUnits=deg  RotationStandardAxis=+Y  RotationAngle=-90  RotationArbitraryAxis=[0 0 1]  FollAlignAxisA=+X  BaseAlignAxisA=+Y  FollAlignAxisB=+Y  BaseAlignAxisB=+Z  RotationSequenceAxes=FollowerAxes  RotationSequence=XYX  RotationSequenceAngles=[0 0 0]  RotationSequenceAnglesUnits=deg  RotationMatrix=[1 0 0; 0 1 0; 0 0 1]
  Rigid Transform1 : sm_lib/Frames and Transforms/Rigid Transform  TranslationMethod=None  TranslationStandardOffset=0  TranslationLengthUnit=m  TranslationStandardAxis=+Z  TranslationCartesianOffset=[0 0 0]  TranslationROffset=0  TranslationROffsetUnits=m  TranslationZOffset=0  TranslationZOffsetUnits=m  TranslationThetaOffset=0  TranslationThetaOffsetUnits=deg  RotationMethod=StandardAxis  RotationAngleUnits=deg  RotationStandardAxis=+Y  RotationAngle=90  RotationArbitraryAxis=[0 0 1]  FollAlignAxisA=+X  BaseAlignAxisA=+Y  FollAlignAxisB=+Y  BaseAlignAxisB=+Z  RotationSequenceAxes=FollowerAxes  RotationSequence=XYX  RotationSequenceAngles=[0 0 0]  RotationSequenceAnglesUnits=deg  RotationMatrix=[1 0 0; 0 1 0; 0 0 1]
  Simulink-PS Converter1 : nesl_utility/Simulink-PS Converter  PhysicalDomain=network_engine_domain  SubClassName=ps_input  LeftPortType=input  RightPortType=output  PseudoPeriodic=off  Frequencies=[]  NoiseDistribution=none  NoiseParameters=[]  Unit=in  AffineConversion=off  FilteringAndDerivatives=provide  SimscapeFilterOrder=1  InputFilterTimeConstant=0.001  UdotUserProvided=0
  Subtract : Sum  Inputs=+-
  F : PMIOPort  Side=Right
  B : PMIOPort  Port=2  Side=Left
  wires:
  Constant1/1 -> Subtract/1
  Constant/1 -> Subtract/2
  Subtract/1 -> Simulink-PS Converter1/1
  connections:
  Prismatic Joint/RConn1 -- Rigid Transform1/LConn1
  Prismatic Joint/LConn2 -- Simulink-PS Converter1/RConn1
  Rigid Transform/RConn1 -- Prismatic Joint/LConn1
  B/RConn1 -- Rigid Transform/LConn1
  Rigid Transform1/RConn1 -- F/RConn1

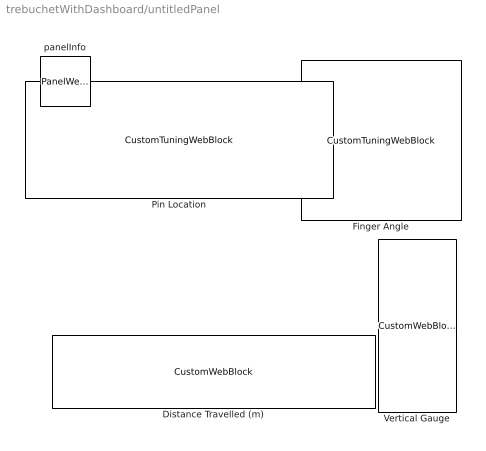
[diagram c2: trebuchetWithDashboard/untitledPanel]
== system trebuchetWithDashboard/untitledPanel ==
  Distance Travelled (m) : CustomWebBlock  Tag=HiddenForWebPanel  PanelInfo="{\"panelId\":\"panelId-7902398d-ba27-4930-a4d3-b1397bd50947\",\"type\":\"panelChild\",\"version\":\"2019b\",\"zIndex\":1500004}"  LabelPosition=Hide  ShowInitialText=on  Configuration="{\"components\":[{\"name\":\"LinearScaleComponent\",\"settings\":{\"bounds\":{\"max\":15,\"min\":0,\"tickInterval\":5},\"internalTickHeightScaleFactor\":1,\"labelColor\":[166,166,166],\"labelFont\":{\"font\":\"Arial\",\"fontSize\":12},\"labelTransparency\":1,\"needleImage\":{\"size\":[273,266],\"src\":\"data:image\\/png;base64,iVBORw0KGgoAAAANSUhEUgAAAREAAAEKCAYAAAA1hWHWAAAACXBIWXMAAA7EAAAOxAGVKw4bAAAAB3RJTUUH5QodCx8Vzkyy5gAAIABJREFUe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"
  Finger Angle : CustomTuningWebBlock  Tag=HiddenForWebPanel  PanelInfo="{\"panelId\":\"panelId-7902398d-ba27-4930-a4d3-b1397bd50947\",\"type\":\"panelChild\",\"version\":\"2019b\",\"zIndex\":1500002}"  LabelPosition=Hide  ShowInitialText=on  Configuration="{\"components\":[{\"name\":\"CircularScaleComponent\",\"settings\":{\"bounds\":{\"max\":60,\"min\":-30,\"tickInterval\":20},\"direction\":\"cw\",\"flipLimits\":0,\"innerRadius\":0.6636618227670849,\"internalTickHeightScaleFactor\":1,\"labelColor\":[166,166,166],\"labelFont\":{\"font\":\"Arial\",\"fontSize\":12},\"labelRadius\":0.8,\"labelTransparency\":0.5,\"minorTickHeightScaleFactor\":0.2,\"needleImage\":{\"size\":[432,144],\"src\":\"data:imag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"
  Pin Location : CustomTuningWebBlock  Tag=HiddenForWebPanel  PanelInfo="{\"panelId\":\"panelId-7902398d-ba27-4930-a4d3-b1397bd50947\",\"type\":\"panelChild\",\"version\":\"2019b\",\"zIndex\":1500008}"  LabelPosition=Hide  ShowInitialText=on  Configuration="{\"components\":[{\"name\":\"LinearScaleComponent\",\"settings\":{\"bounds\":{\"max\":10,\"min\":0,\"tickInterval\":0.1},\"internalTickHeightScaleFactor\":0.5,\"labelColor\":[38,38,38],\"labelFont\":{\"font\":\"Arial\",\"fontSize\":12},\"labelTransparency\":0,\"needleImage\":{\"size\":[960,240],\"src\":\"data:image\\/svg+xml;base64,PHN2ZyB3aWR0aD0iOTYwIiBoZWlnaHQ9IjI0MCIgeG1sbnM9Imh0dHA6Ly93d3cudzMub3JnLzIwMDAvc3ZnIiB4bWxuczp4bGluaz0i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"
  Vertical Gauge : CustomWebBlock  Tag=HiddenForWebPanel  PanelInfo="{\"panelId\":\"panelId-7902398d-ba27-4930-a4d3-b1397bd50947\",\"type\":\"panelChild\",\"version\":\"2019b\",\"zIndex\":1500006}"  LabelPosition=Hide  ShowInitialText=on  Configuration="{\"components\":[{\"name\":\"LinearScaleComponent\",\"settings\":{\"bounds\":{\"max\":8,\"min\":0,\"tickInterval\":\"auto\"},\"internalTickHeightScaleFactor\":0.5,\"labelColor\":[128,128,128],\"labelFont\":{\"font\":\"Arial\",\"fontSize\":12},\"labelTransparency\":1,\"needleImage\":{\"size\":[273,266],\"src\":\"data:image\\/png;base64,iVBORw0KGgoAAAANSUhEUgAAAREAAAEKCAYAAAA1hWHWAAAACXBIWXMAAA7EAAAOxAGVKw4bAAAAB3RJTUUH5QodCx8Vzkyy5gAAIAB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"
  panelInfo : PanelWebBlock  Tag=HiddenForWebPanel  PanelInfo="{\"compacted\":false,\"height\":386,\"isActiveTab\":true,\"left\":14,\"name\":\"Panel\",\"panelId\":\"panelId-7902398d-ba27-4930-a4d3-b1397bd50947\",\"tabIndex\":0,\"tabbedSetId\":\"tabbedSet5447478774\",\"top\":121,\"type\":\"panel\",\"version\":\"2019b\",\"visible\":true,\"width\":454,\"zIndex\":1500002}"  PanelSnapshot=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

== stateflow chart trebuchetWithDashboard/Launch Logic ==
  state Engaged
    mode = 0;
  state Disengaged
    mode = -1;
  (default) -> Engaged
  Engaged -> Disengaged : [(finang + u + theta0) < 0]
  data: u input; mode output; finang parameter; theta0 constant double =122.7042
